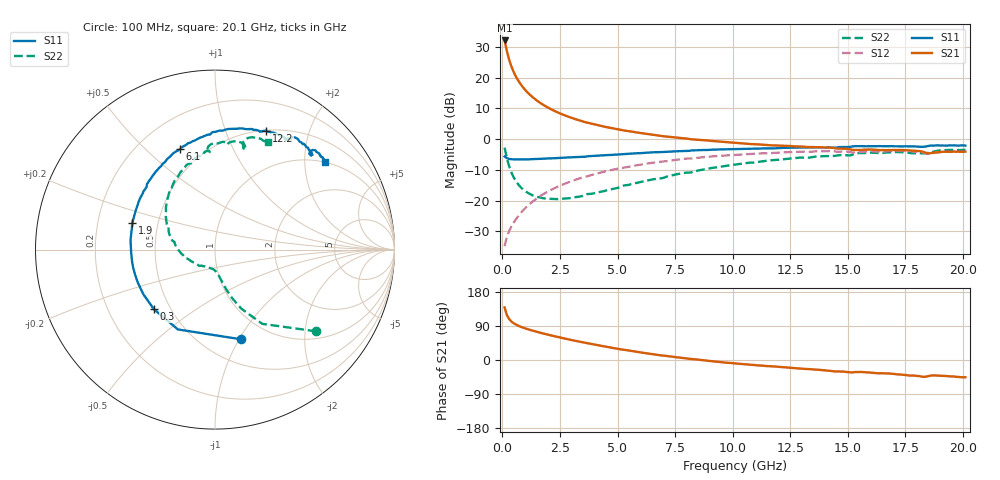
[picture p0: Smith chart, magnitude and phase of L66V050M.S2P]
!  Infineon Technologies AG
! BFR380L3 , PF131585-7, No.6, Th 09.10.01, soldered on pcb-board, measured with PP GSG850
!  Vce=6.0 V,  Ic=50.0 mA
! Common Emitter S-Parameters:  15. November 2001
#  GHz  S  MA  R  50
! f  S11  S21  S12  S22
! GHz  Mag  Ang  Mag  Ang  Mag  Ang  Mag  Ang
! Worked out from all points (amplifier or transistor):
!   201 points, 100 MHz to 20.1 GHz, reference 50 ohm
!   highest |S21| = 32.1 dB at 100 MHz (marker M1)
!   |S21| within 3 dB of that: start of sweep to 185.2 MHz
!   unconditionally stable (mu >= 1): 987.9 MHz to 4.293 GHz
!   at 3.4 GHz: K = 1.02, MAG = 8.4 dB, |S12| = -12.7 dB
!   at 10.1 GHz: K = 0.94, MSG = 1.9 dB, |S12| = -5.1 dB
!   at 20.1 GHz: K = 0.99, MSG = 0.0 dB, |S12| = -4.0 dB
!   S11 on the Smith chart (normalised r, x): 100 MHz: 0.74, -1.02; 300 MHz: 0.41, -0.35; 1.9 GHz: 0.36, +0.14; 6.1 GHz: 0.37, +0.64; 12.2 GHz: 0.50, +1.40; 20.1 GHz: 0.99, +2.52
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0.1  0.521 -73.7  40.19 138.8  0.01816 63.5  0.7256 -38.9
0.2  0.4905 -115.0  26.8 118.2  0.02596 56.9  0.4905 -57.5
0.3  0.4757 -135.6  19.35 107.8  0.03237 57.9  0.3603 -66.0
0.4  0.4703 -148.0  15 101.3  0.03808 59.7  0.2844 -70.7
0.5  0.4678 -156.5  12.19 96.8  0.04415 62.2  0.2368 -73.8
0.6  0.4668 -162.5  10.25 93.3  0.05021 63.9  0.2049 -76.0
0.7  0.467 -167.4  8.844 90.3  0.05632 65.0  0.1817 -77.9
0.8  0.4669 -171.5  7.772 87.7  0.06289 66.2  0.1649 -79.5
1  0.4675 -178.1  6.27 83.4  0.07579 67.3  0.142 -82.4
1.2  0.4699 176.5  5.255 79.5  0.08879 67.8  0.1281 -85.7
1.5  0.4745 169.9  4.24 74.3  0.1087 67.7  0.1155 -90.7
1.9  0.4834 162.4  3.388 68.1  0.1352 66.5  0.1081 -98.4
2.6  0.4962 150.9  2.526 58.1  0.181 63.4  0.1075 -113.8
3.5  0.5157 138.1  1.933 46.5  0.239 58.1  0.1199 -131.5
4.6  0.551 124.7  1.546 33.9  0.3067 51.2  0.1492 -154.8
6.1  0.5937 109.1  1.239 19.1  0.3899 41.1  0.2049 -179.7
6.8  0.6139 102.5  1.14 13.0  0.4262 36.0  0.2294 170.0
10.1  0.6899 78.0  0.8671 -9.1  0.5549 14.2  0.3853 133.6
12.2  0.7222 66.6  0.781 -19.1  0.6099 1.0  0.4721 114.0
13.5  0.7313 60.2  0.7435 -24.9  0.6274 -7.1  0.5117 103.7
16.8  0.7665 47.9  0.6637 -35.6  0.6357 -23.6  0.6087 81.0
20.1  0.7852 38.5  0.6265 -45.5  0.6279 -37.6  0.6688 63.9
